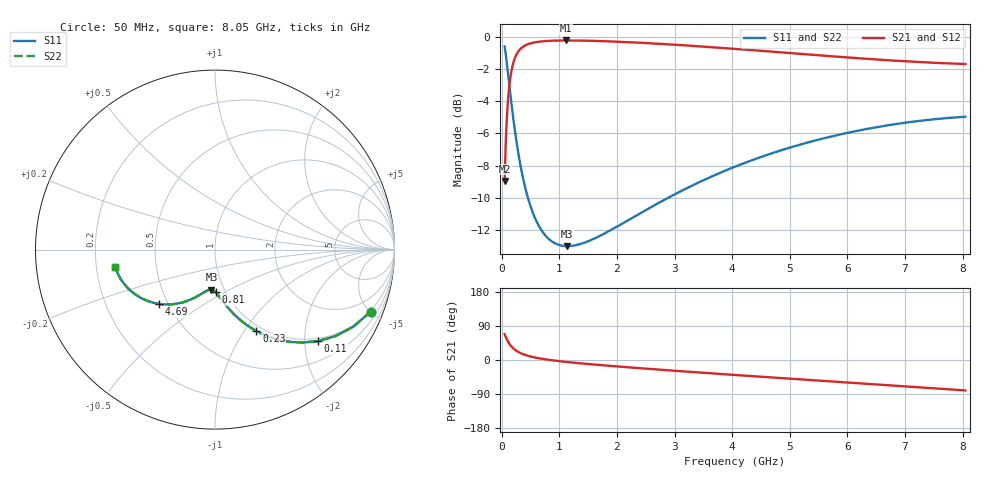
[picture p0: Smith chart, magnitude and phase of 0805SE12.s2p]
! AVX Thin Film Operation		Date: August 2001
! Description: Accu-P® Series, Thin Film, SMD, RF Capacitor
! Part Number: 08055J120FBT
! 50 MHz  -  8.05 GHz
! Serial Measurements
# mhz S db R 50
!	S11		S21		S12		S22
!	dB	Phase	dB	Phase	dB	Phase	dB	Phase
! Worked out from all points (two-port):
!   401 points, 50 MHz to 8.05 GHz, reference 50 ohm
!   highest |S21| = -0.23 dB at 1.11 GHz (marker M1); lowest = -9.0 dB at 50 MHz (marker M2)
!   |S21| within 3 dB of the highest: 126.6 MHz to end of sweep
!   lowest |S11| = -13.0 dB at 1.13 GHz (marker M3), VSWR 1.58, Z = 43.6 - j20.4 ohm
!   |S11| at or under -10 dB: 454.6 MHz to 2.889 GHz (2.435 GHz wide, 146 % of centre)
!   |S22| runs from -13.0 to -0.6 dB; largest |S21 - S12| = 0
!   S11 on the Smith chart (normalised r, x): 50 MHz: 0.93, -5.05; 110 MHz: 0.93, -2.31; 230 MHz: 0.93, -1.14; 810 MHz: 0.90, -0.45; 4.69 GHz: 0.45, -0.33; 8.05 GHz: 0.28, -0.08
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50  -0.59 -21.7  -8.95 68.3  -8.95 68.3  -0.59 -21.7
70  -1.09 -29.2  -6.55 60.8  -6.55 60.8  -1.09 -29.2
110  -2.29 -41.6  -3.87 48.4  -3.87 48.4  -2.29 -41.6
130  -2.93 -46.6  -3.09 43.4  -3.09 43.4  -2.93 -46.6
170  -4.18 -54.6  -2.09 35.4  -2.09 35.4  -4.18 -54.6
190  -4.77 -57.8  -1.76 32.2  -1.76 32.2  -4.77 -57.8
230  -5.87 -63.1  -1.30 26.9  -1.30 26.9  -5.87 -63.1
270  -6.84 -67.2  -1.01 22.7  -1.01 22.7  -6.84 -67.2
310  -7.69 -70.6  -0.81 19.4  -0.81 19.4  -7.69 -70.6
430  -9.68 -77.7  -0.50 12.2  -0.50 12.2  -9.68 -77.7
610  -11.51 -84.3  -0.32 5.6  -0.32 5.6  -11.51 -84.3
810  -12.54 -89.3  -0.25 0.7  -0.25 0.7  -12.54 -89.3
1110  -13.00 -94.8  -0.23 -4.9  -0.23 -4.9  -13.00 -94.8
1130  -13.01 -95.1  -0.23 -5.2  -0.23 -5.2  -13.01 -95.1
1390  -12.85 -99.0  -0.23 -9.1  -0.23 -9.1  -12.85 -99.0
2010  -11.77 -107.0  -0.30 -17.1  -0.30 -17.1  -11.77 -107.0
2730  -10.31 -115.3  -0.43 -25.4  -0.43 -25.4  -10.31 -115.3
4050  -8.07 -129.4  -0.75 -39.5  -0.75 -39.5  -8.07 -129.4
4690  -7.23 -136.0  -0.92 -46.1  -0.92 -46.1  -7.23 -136.0
5390  -6.49 -143.1  -1.11 -53.2  -1.11 -53.2  -6.49 -143.1
6730  -5.48 -156.6  -1.46 -66.7  -1.46 -66.7  -5.48 -156.6
8050  -4.97 -170.1  -1.69 -80.3  -1.69 -80.3  -4.97 -170.1
